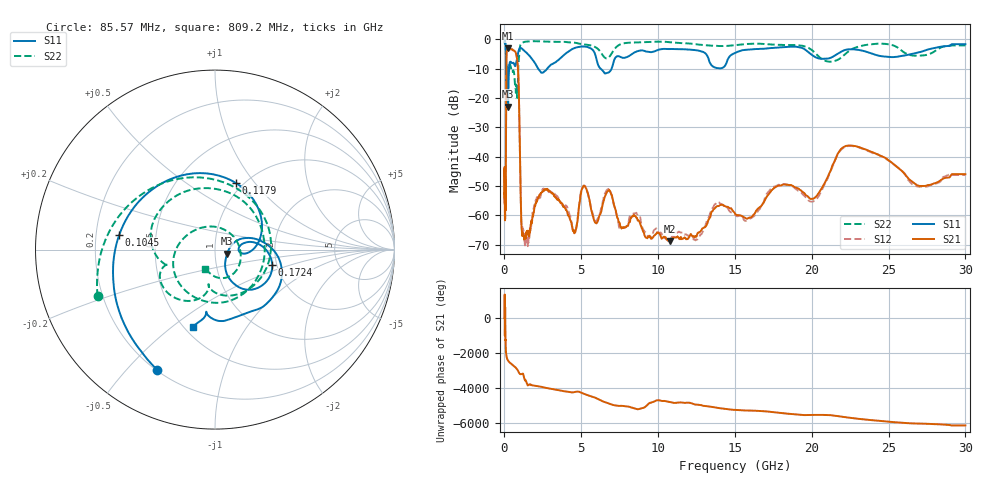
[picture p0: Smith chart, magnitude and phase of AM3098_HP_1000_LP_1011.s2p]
! Date/Time: Thu, Feb 28, 2019 8:40 AM
! Network Analyzer: Agilent Technologies E8364B Rev: A.07.50.67
! Sweep from 0.010 to 30.000 GHz, 1601 Points, Sweep Type: LOG
! Power Supply: 5.023 V, 0.002 A
# Hz S DB R 50
!freq MagS11 AngS11 MagS21 AngS21 MagS12 AngS12 MagS22 AngS22
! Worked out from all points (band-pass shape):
!   1601 points, 10 MHz to 30 GHz, reference 50 ohm
!   highest |S21| = -3.08 dB at 242.3 MHz (marker M1); lowest = -68.9 dB at 10.76 GHz (marker M2)
!   |S21| within 3 dB of the highest: 128.1 MHz to 805.3 MHz (677.3 MHz wide, 145 % of centre)
!   lowest |S11| = -22.9 dB at 238.7 MHz (marker M3), VSWR 1.15, Z = 57.2 - j2.56 ohm
!   |S11| at or under -10 dB: 191.6 MHz to 300.6 MHz (109 MHz wide, 44.3 % of centre); 2.193 GHz to 2.78 GHz (586.7 MHz wide, 23.6 % of centre); 6.263 GHz to 6.971 GHz (708.3 MHz wide, 10.7 % of centre)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
!   |S22| runs from -20.0 to -0.6 dB; largest |S21 - S12| = 0.01
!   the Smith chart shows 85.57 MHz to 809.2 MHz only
!   S11 on the Smith chart (normalised r, x): 85.57 MHz: 0.20, -0.61; 104.5 MHz: 0.30, +0.07; 117.9 MHz: 0.93, +0.81; 172.4 MHz: 1.89, -0.37; 809.2 MHz: 0.55, -0.59
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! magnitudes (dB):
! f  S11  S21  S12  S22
! 10 MHz  -0.4  -44.4  -43.8  -0.6
! 38.04 MHz  -0.5  -61.2  -60.4  -1.0
! 49.1 MHz  -0.8  -48.5  -51.6  -1.3
! 85.57 MHz  -2.6  -53.5  -53.7  -3.0
! 104.5 MHz  -5.4  -27.9  -28.1  -6.8
! 117.9 MHz  -8.2  -11.3  -11.3  -10.3
! 144.7 MHz  -16.8  -4.3  -4.2  -13.2
! 172.4 MHz  -9.6  -3.8  -3.8  -9.2
! 238.7 MHz  -22.9  -3.1  -3.0  -11.2
! 242.3 MHz  -22.6  -3.1  -3.0  -11.2
! 550.5 MHz  -8.0  -3.7  -3.6  -10.6
! 809.2 MHz  -7.0  -6.2  -6.2  -18.4
! 921.7 MHz  -3.9  -15.0  -15.0  -7.6
! 1.143 GHz  -3.2  -66.6  -64.4  -1.2
! 2.084 GHz  -9.0  -55.6  -54.4  -0.6
! 4.548 GHz  -3.0  -66.1  -66.2  -1.1
! 5.206 GHz  -2.4  -50.1  -50.1  -1.7
! 7.926 GHz  -6.1  -64.0  -63.8  -1.2
! 10.76 GHz  -3.3  -68.9  -69.1  -1.0
! 20.1 GHz  -5.6  -54.4  -55.3  -4.0
! 22.56 GHz  -3.4  -36.2  -36.4  -3.5
! 30 GHz  -1.6  -46.0  -46.3  -2.1
